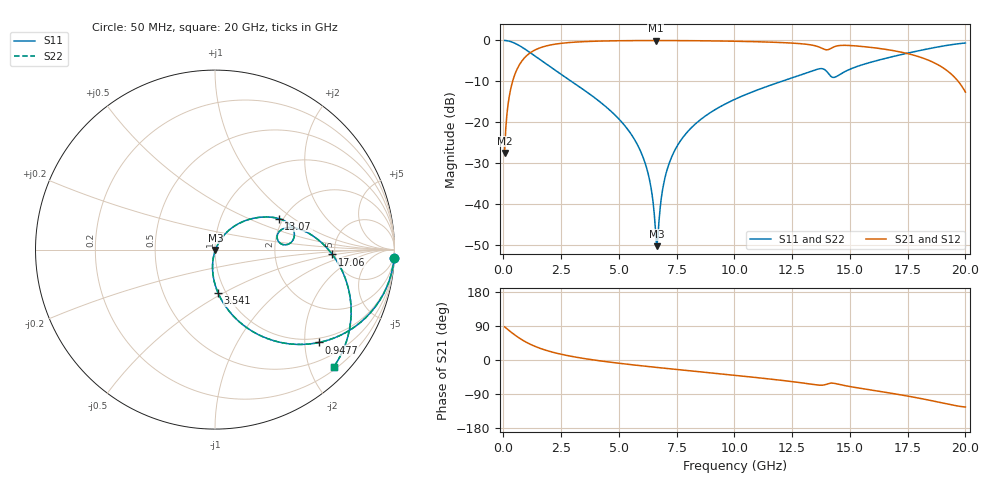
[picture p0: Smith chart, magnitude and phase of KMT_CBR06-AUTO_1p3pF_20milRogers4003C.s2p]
! Data measured by Modelithics Inc. support@modelithics.com 813-866-6335
! KEMET CBR06-AUTO 1.3pF, Pad Width= 0.851mm, Pad Length= 0.64mm, Pad Gap= 0.62mm, 20mil Rogers 4003C substrate Data, January 2022
# hz S ma R 50
! 2 Port Network Data from SP1.SP block
! freq  magS11  angS11  magS21  angS21  magS12  angS12  magS22  angS22
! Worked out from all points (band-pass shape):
!   401 points, 50 MHz to 20 GHz, reference 50 ohm
!   highest |S21| = -0.03 dB at 6.584 GHz (marker M1); lowest = -27.6 dB at 50 MHz (marker M2)
!   |S21| within 3 dB of the highest: 1.161 GHz to 17.35 GHz (16.19 GHz wide, 175 % of centre)
!   lowest |S11| = -50.4 dB at 6.633 GHz (marker M3), VSWR 1.01, Z = 50.3 - j0.161 ohm
!   |S11| at or under -10 dB: 2.938 GHz to 12.06 GHz (9.12 GHz wide, 122 % of centre)
!   |S22| runs from -50.4 to 0.0 dB; largest |S21 - S12| = 0
!   S11 on the Smith chart (normalised r, x): 50 MHz: 1, -45; 947.8 MHz: 0.89, -2.33; 3.541 GHz: 0.92, -0.47; 13.07 GHz: 1.89, +0.78; 17.06 GHz: 4.74, -0.45; 20 GHz: 0.25, -2.41
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5e7  0.9991 -2.5  0.04177 87.4  0.04177 87.4  0.9991 -2.5
3.4925e8  0.9595 -17.4  0.2809 72.6  0.2809 72.6  0.9595 -17.4
9.4775e8  0.7775 -41.7  0.6277 48.2  0.6277 48.2  0.7775 -41.7
1.94525e9  0.4925 -66.1  0.8685 23.7  0.8685 23.7  0.4925 -66.1
3.391625e9  0.258 -84.6  0.9638 4.9  0.9638 4.9  0.258 -84.6
3.54125e9  0.2409 -86.0  0.9681 3.4  0.9681 3.4  0.2409 -86.0
5.785625e9  0.05383 -101.1  0.9956 -14.1  0.9956 -14.1  0.05383 -101.1
6.284375e9  0.0221 -99.9  0.9967 -17.3  0.9967 -17.3  0.0221 -99.9
6.583625e9  0.004679 -70.3  0.9968 -19.3  0.9968 -19.3  0.004679 -70.3
6.6335e9  0.003023 -31.9  0.9968 -19.6  0.9968 -19.6  0.003023 -31.9
6.73325e9  0.006084 40.5  0.9968 -20.2  0.9968 -20.2  0.006084 40.5
7.0325e9  0.02308 60.3  0.9964 -22.1  0.9964 -22.1  0.02308 60.3
7.581125e9  0.05432 61.1  0.9951 -25.5  0.9951 -25.5  0.05432 61.1
8.52875e9  0.107 56.8  0.9905 -31.3  0.9905 -31.3  0.107 56.8
1.0025e10  0.1904 48.3  0.9772 -40.5  0.9772 -40.5  0.1904 48.3
1.306738e10  0.3953 25.9  0.9007 -61.5  0.9007 -61.5  0.3953 25.9
1.336662e10  0.4235 21.8  0.876 -64.1  0.876 -64.1  0.4235 21.8
1.431425e10  0.3525 11.0  0.8353 -61.5  0.8353 -61.5  0.3525 11.0
1.670825e10  0.6195 1.3  0.7645 -86.9  0.7645 -86.9  0.6195 1.3
1.705738e10  0.6541 -2.4  0.7341 -90.4  0.7341 -90.4  0.6541 -2.4
1.890275e10  0.8414 -25.7  0.4871 -112.0  0.4871 -112.0  0.8414 -25.7
2e10  0.9297 -44.6  0.2331 -124.0  0.2331 -124.0  0.9297 -44.6
